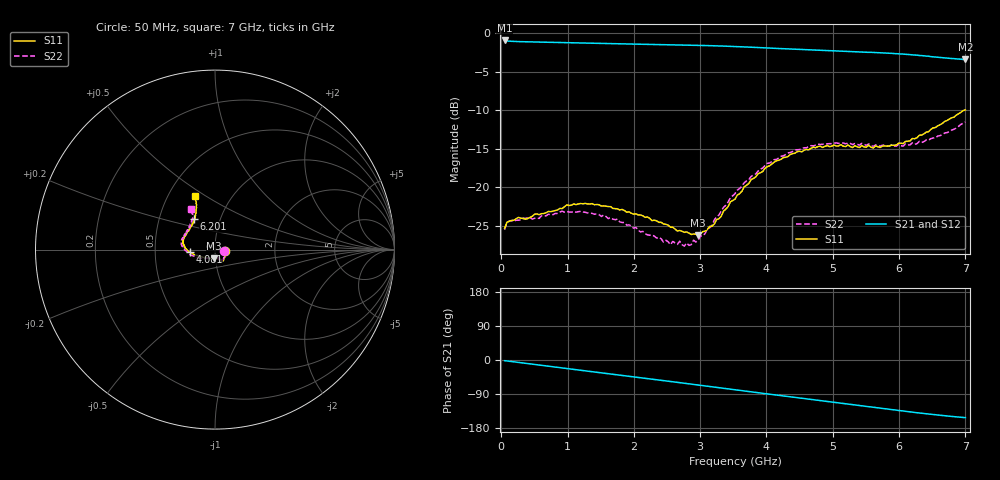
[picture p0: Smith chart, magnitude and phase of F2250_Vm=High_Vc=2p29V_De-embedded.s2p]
! Integrated Device Technology
! Corporate Headquarters
! 6024 Silver Creek Valley Road
! San Jose, CA 95138  USA
! Phone:  1-408-284-8200
! Toll Free:  1-800-223-1366
! Webpage:  http://www.idt.com/
! Timing and RF Division
! 515 Groton Road, Suite 102
! Westford, MA 01886-6024
! Device:  F2250
! Description: Voltage Variable RF Attenuator
! Frequency:  50.0 -  6000.00 MHz
! Package:  3x3 mm Thin QFN Plastic Package: 16 pin
! Ports:  2 RF, 3 DC
!  Pin  1  = GND
!  Pin  2  = NC
!  Pin  3  = RF1  = Port 1
!  Pin  4  = NC
!  Pin  5  = GND
!  Pin  6  = GND
!  Pin  7  = GND
!  Pin  8  = GND
!  Pin  9  = NC
!  Pin 10  = RF2  = Port 2
!  Pin 11  = NC
!  Pin 12  = GND
!  Pin 13  = GND
!  Pin 14  = VCNTRL
!  Pin 15  = VDD
!  Pin 16  = VMODE
! Vcntrl:  2.290 Volts
! Vmode:  +3.300 Volts
! Vdd:  +3.30  Volts
! Current:  1.317 mA
! Data:  The device was measured on a the F2250 evaluation board which has
!  individual transmission lines to the RF pins.  Data was collected
!  using a calibrated network analyzer.  The evaluation board was
!  de-embedded using a TRL calibration technique.
!  The reference plane is the edge of the package pin.
! Misc:  SN 10
!  Action Tracker AT0258
! Date Measured:  2014-11-26
! Date:  2015-10-15  MJV
! Note:
!  Integrated Device Technology supplies this data as a sample of measured
!  data at the package pin for this product.  Your particular data for this
!  product may vary.
!  Data was taken at 25 degrees C.
!  Integrated Device Technology reserves the right to change this data at anytime.
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# GHz S dB R 50
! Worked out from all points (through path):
!   201 points, 50 MHz to 7 GHz, reference 50 ohm
!   highest |S21| = -0.91 dB at 50 MHz (marker M1); lowest = -3.4 dB at 7 GHz (marker M2)
!   group delay of S21, straight-line fit = 61.1 ps
!   lowest |S11| = -26.3 dB at 2.969 GHz (marker M3), VSWR 1.10, Z = 49.3 - j4.78 ohm
!   |S11| at or under -10 dB: start of sweep to 6.983 GHz
!   |S22| runs from -27.7 to -11.5 dB; largest |S21 - S12| = 0.0019
!   S11 on the Smith chart (normalised r, x): 50 MHz: 1.11, -0.02; 4.081 GHz: 0.75, -0.02; 6.201 GHz: 0.75, +0.27; 7 GHz: 0.68, +0.45
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0.05  -25.37 -10.3  -0.91 -1.8  -0.91 -1.8  -25.53 -10.7
0.1195  -24.46 -10.0  -1.00 -3.2  -1.00 -3.2  -24.41 -8.7
0.57125  -23.58 -30.7  -1.12 -13.3  -1.12 -13.3  -24.07 -31.0
0.91875  -22.79 -49.2  -1.19 -21.0  -1.19 -21.1  -23.13 -50.5
1.2315  -22.17 -57.0  -1.26 -27.9  -1.26 -27.9  -23.25 -61.0
1.75275  -22.83 -63.9  -1.35 -39.1  -1.35 -39.1  -24.16 -67.5
2.37825  -24.59 -63.7  -1.44 -52.8  -1.44 -52.8  -26.54 -67.3
2.552  -25.22 -68.5  -1.46 -56.7  -1.46 -56.7  -27.49 -73.7
2.691  -25.64 -76.3  -1.49 -59.8  -1.49 -59.8  -27.04 -81.3
2.7605  -25.88 -78.4  -1.50 -61.3  -1.50 -61.3  -27.69 -85.8
2.969  -26.26 -96.1  -1.54 -66.0  -1.54 -66.0  -26.95 -104.8
3.21225  -24.81 -126.1  -1.60 -71.5  -1.60 -71.5  -24.28 -129.8
3.525  -21.56 -151.4  -1.70 -78.5  -1.70 -78.6  -20.85 -148.4
3.76825  -19.01 -163.8  -1.79 -84.0  -1.79 -84.0  -18.61 -159.4
4.081  -17.00 -175.0  -1.92 -91.0  -1.92 -91.0  -16.66 -171.2
4.4285  -15.58 176.6  -2.05 -98.6  -2.05 -98.6  -15.15 178.9
4.7065  -14.81 169.6  -2.15 -104.8  -2.15 -104.8  -14.64 173.1
5.054  -14.65 161.4  -2.28 -112.5  -2.27 -112.5  -14.24 166.1
5.85325  -14.63 135.5  -2.58 -130.0  -2.58 -130.1  -14.65 147.3
6.20075  -13.68 123.9  -2.78 -137.7  -2.79 -137.8  -14.23 138.3
6.54825  -12.24 115.9  -3.06 -144.7  -3.06 -144.8  -13.57 126.9
7  -9.95 111.0  -3.38 -152.1  -3.39 -152.2  -11.54 120.7
